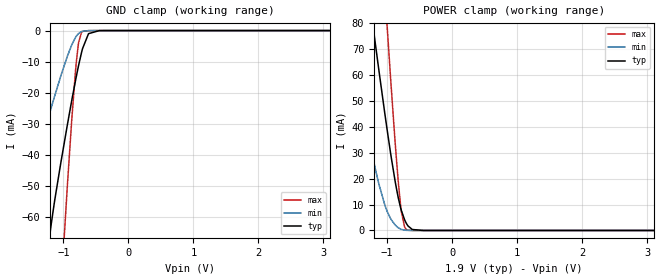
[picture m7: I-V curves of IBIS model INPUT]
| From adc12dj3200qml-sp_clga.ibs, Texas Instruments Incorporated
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[Model]   INPUT
Model_type   Input
Vinl = 0.45
Vinh = 0.7
|   typ   min   max
C_comp   0.62p   0.51p   0.71p
[Voltage Range]   1.9   1.8   2
[Temperature Range]   25   125   -40
[Power Clamp Reference]   1.9   1.8   2
[GND Clamp Reference]   0   0   0
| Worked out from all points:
|   GND clamp passes 1 mA (typ) near -0.61 V on its own axis
|   POWER clamp passes 1 mA (typ) near -0.64 V on its own axis
[GND Clamp]
|   Voltage   I(typ)   I(min)   I(max)
-1.8V     -213.8mA   -95.1mA    -502.1mA
-1.616V   -163.5mA   -66.03mA   -393.9mA
-1.4V     -107.1mA   -40.97mA   -268.6mA
-1.195V   -63.81mA   -25.52mA   -155mA
-1.033V   -41.99mA   -14.29mA   -82.69mA
-936mV    -30.19mA   -8.176mA   -49.49mA
-801mV    -14.91mA   -1.832mA   -10.44mA
-763.2mV  -11.06mA   -906.3uA   -3.733mA
-720mV    -7.113mA   -343.3uA   -610uA
-612mV    -992.3uA   -21.03uA   -2.371uA
-444.6mV  -6.592uA   -208.8nA   0A
3.6V      0A         0A         0A
[POWER Clamp]
|   Voltage   I(typ)   I(min)   I(max)
-1.8V     194.1mA    101.9mA    402.9mA
-1.4V     114.5mA    50.02mA    238.7mA
-1.287V   92.46mA    36.09mA    192.7mA
-1.184V   72.81mA    24.22mA    151.4mA
-1.001V   39.17mA    7.504mA    79.47mA
-871.2mV  18.34mA    2.033mA    32.53mA
-822.6mV  12.06mA    973.6uA    17.5mA
-779.4mV  7.657mA    417.4uA    7.2mA
-730.8mV  4.154mA    133.6uA    1.361mA
-676.8mV  1.722mA    33.4uA     107.6uA
-444.6mV  2.42uA     41.99nA    0A
3.6V      0A         0A         0A
